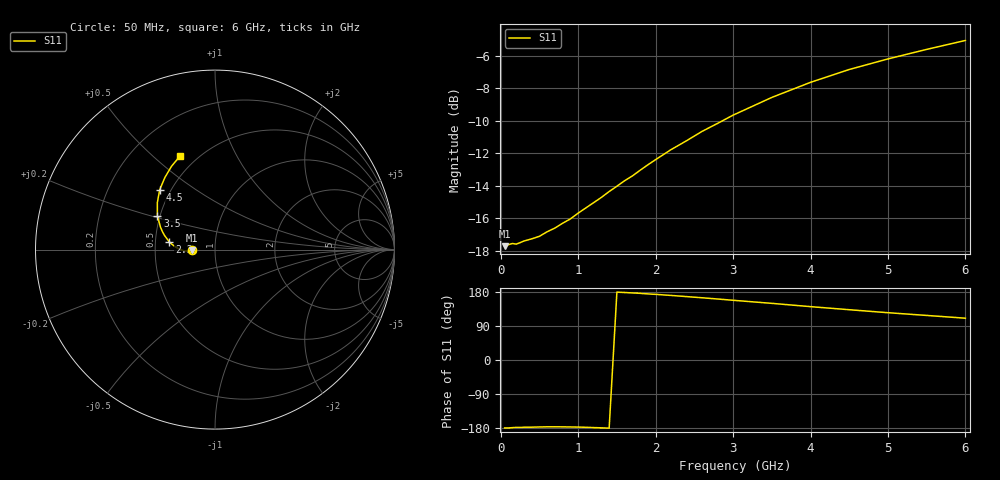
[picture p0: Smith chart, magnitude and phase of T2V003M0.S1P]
! SIEMENS Discrete & RF Semiconductors
! BAS70-04W
! Si Schottky Diode in SOT323
! IF = 3 mA
! S-Parameters:  November  1997
# GHz  S  MA  R  50
!  f  S11
! GHz  MAG  ANG
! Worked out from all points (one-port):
!   34 points, 50 MHz to 6 GHz, reference 50 ohm
!   lowest |S11| = -17.7 dB at 50 MHz (marker M1), VSWR 1.30, Z = 38.5 - j0.142 ohm
!   |S11| at or under -10 dB: start of sweep to 2.867 GHz
!   S11 on the Smith chart (normalised r, x): 50 MHz: 0.77, -0.00; 2.2 GHz: 0.59, +0.05; 3.5 GHz: 0.48, +0.21; 4.5 GHz: 0.44, +0.37; 6 GHz: 0.41, +0.62
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0.05  0.1301 -179.2
0.1  0.1315 -179.3
0.15  0.1326 -178.5
0.2  0.132 -177.9
0.25  0.1333 -178.1
0.3  0.1349 -177.4
0.5  0.1395 -176.7
0.6  0.144 -176.3
0.7  0.1479 -176.2
0.8  0.153 -176.4
0.9  0.1578 -176.7
1  0.1643 -177.0
1.3  0.1837 -179.0
1.6  0.2067 178.1
1.7  0.2138 177.0
1.8  0.2226 175.9
2  0.2399 173.2
2.2  0.2576 170.4
2.4  0.2743 167.3
2.6  0.2931 164.2
2.8  0.3101 161.0
3  0.3287 157.6
3.5  0.3726 149.5
4  0.4146 140.8
4.5  0.454 132.7
5  0.4893 124.8
5.5  0.5234 117.6
6  0.5576 110.3
